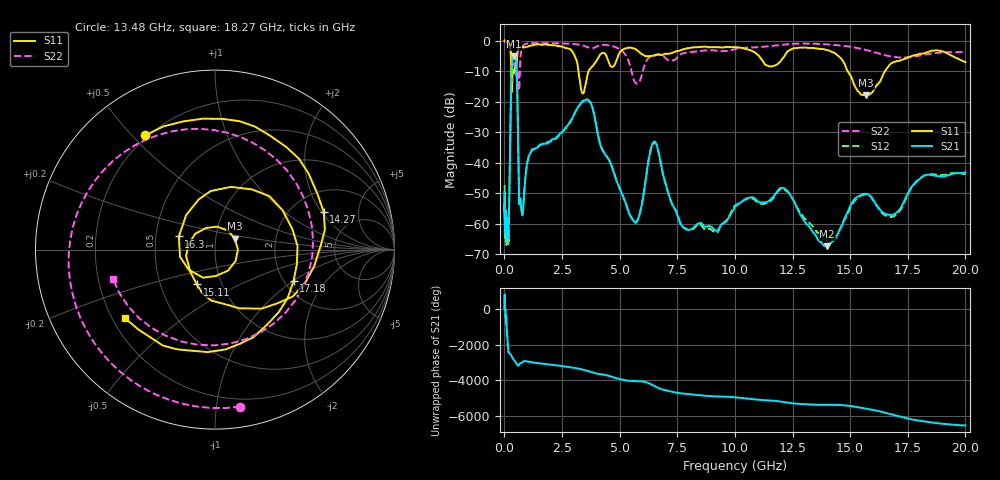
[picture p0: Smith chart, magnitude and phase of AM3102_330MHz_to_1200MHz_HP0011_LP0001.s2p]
! Date/Time: Tue, Sep 11, 2018 5:11 PM
! Network Analyzer: Agilent Technologies E8362B Rev: A.07.50.63
! Sweep from 0.010 to 20.000 GHz, 1601 Points, Sweep Type: LOG
! Power Supply: 4.950 V, 0.001 A
# Hz S DB R 50
!freq MagS11 AngS11 MagS21 AngS21 MagS12 AngS12 MagS22 AngS22
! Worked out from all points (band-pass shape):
!   1601 points, 10 MHz to 20 GHz, reference 50 ohm
!   highest |S21| = -5.22 dB at 406.7 MHz (marker M1); lowest = -67.4 dB at 14.01 GHz (marker M2)
!   |S21| within 3 dB of the highest: 321.2 MHz to 522.3 MHz (201.1 MHz wide, 47.7 % of centre)
!   lowest |S11| = -18.0 dB at 15.7 GHz (marker M3), VSWR 1.29, Z = 62 + j7.63 ohm
!   |S11| at or under -10 dB: 298.8 MHz to 360.7 MHz (61.96 MHz wide, 18.8 % of centre); 3.21 GHz to 3.654 GHz (444.4 MHz wide, 12.9 % of centre); 14.89 GHz to 16.51 GHz (1.621 GHz wide, 10.3 % of centre)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
!   |S22| runs from -16.2 to -0.2 dB; largest |S21 - S12| = 0.0074
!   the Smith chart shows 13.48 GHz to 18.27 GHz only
!   S11 on the Smith chart (normalised r, x): 13.48 GHz: 0.19, +0.54; 14.27 GHz: 2.95, +2.11; 15.11 GHz: 0.76, -0.31; 16.3 GHz: 0.66, +0.10; 17.18 GHz: 2.24, -1.01; 18.27 GHz: 0.25, -0.32
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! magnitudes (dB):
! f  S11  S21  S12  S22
! 10 MHz  0.0  -53.5  -47.3  -0.2
! 35.55 MHz  0.0  -58.4  -61.0  -0.4
! 126.4 MHz  -0.4  -62.1  -62.4  -0.8
! 186.6 MHz  -1.0  -59.2  -65.2  -1.2
! 308.7 MHz  -14.3  -10.6  -10.6  -6.8
! 406.7 MHz  -10.7  -5.2  -5.3  -8.0
! 447.2 MHz  -9.2  -5.6  -5.6  -7.3
! 761.4 MHz  -2.2  -56.7  -56.8  -2.5
! 1.59 GHz  -1.4  -34.0  -34.1  -0.8
! 3.634 GHz  -10.4  -19.6  -19.4  -2.3
! 5.652 GHz  -2.7  -59.4  -59.5  -13.5
! 6.518 GHz  -4.9  -33.1  -33.3  -4.7
! 7.882 GHz  -2.6  -61.9  -61.7  -4.0
! 13.48 GHz  -2.5  -63.5  -62.0  -1.0
! 14.01 GHz  -3.1  -67.4  -65.5  -1.3
! 14.27 GHz  -3.9  -65.7  -64.5  -1.4
! 15.11 GHz  -13.2  -52.8  -53.3  -2.2
! 15.7 GHz  -18.0  -50.2  -50.5  -3.1
! 16.3 GHz  -13.4  -55.5  -55.9  -4.3
! 17.18 GHz  -6.5  -55.0  -55.5  -5.6
! 18.27 GHz  -4.0  -44.1  -44.1  -4.6
! 20 GHz  -7.0  -43.3  -43.8  -3.8
